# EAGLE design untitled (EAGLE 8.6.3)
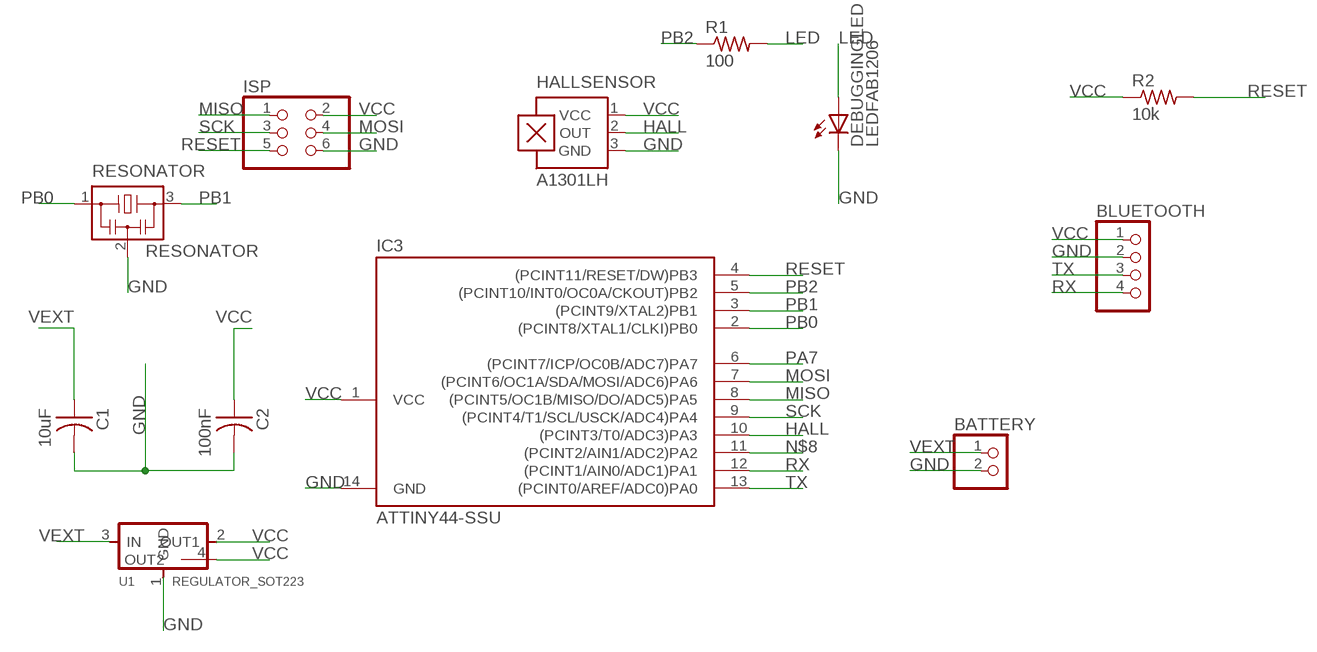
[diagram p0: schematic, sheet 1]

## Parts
BATTERY  PINHD-1X2  [1X02]
BLUETOOTH  PINHD-1X4  [1X04]
C1  10uF  CAP-US1206FAB  [C1206FAB]
C2  100nF  CAP-US1206FAB  [C1206FAB]
DEBUGGINGLED  LEDFAB1206  [LED1206FAB]
HALLSENSOR  A1301LH  [SOT23-W]
IC3  ATTINY44-SSU  [SOIC14]
ISP  PINHD-2X3-SMD  [2X03SMD]
R1  100  RES-US1206FAB  [R1206FAB]
R2  10k  RES-US1206FAB  [R1206FAB]
RESONATOR  RESONATOR  [EFOBM]
U1  REGULATOR_SOT223  [SOT223]

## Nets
GND: BATTERY.2 BLUETOOTH.2 C1.2 C2.2 DEBUGGINGLED.2(C) HALLSENSOR.3(GND) IC3.14(GND) ISP.6 RESONATOR.2 U1.1(GND)
HALL: HALLSENSOR.2(OUT) IC3.10((PCINT3/T0/ADC3)PA3)
LED: DEBUGGINGLED.1(A) R1.2
MISO: IC3.8((PCINT5/OC1B/MISO/DO/ADC5)PA5) ISP.1
MOSI: IC3.7((PCINT6/OC1A/SDA/MOSI/ADC6)PA6) ISP.4
N$8: IC3.11((PCINT2/AIN1/ADC2)PA2)
PA7: IC3.6((PCINT7/ICP/OC0B/ADC7)PA7)
PB0: IC3.2((PCINT8/XTAL1/CLKI)PB0) RESONATOR.1
PB1: IC3.3((PCINT9/XTAL2)PB1) RESONATOR.3
PB2: IC3.5((PCINT10/INT0/OC0A/CKOUT)PB2) R1.1
RESET: IC3.4((PCINT11/RESET/DW)PB3) ISP.5 R2.2
RX: BLUETOOTH.4 IC3.12((PCINT1/AIN0/ADC1)PA1)
SCK: IC3.9((PCINT4/T1/SCL/USCK/ADC4)PA4) ISP.3
TX: BLUETOOTH.3 IC3.13((PCINT0/AREF/ADC0)PA0)
VCC: BLUETOOTH.1 C2.1 HALLSENSOR.1(VCC) IC3.1(VCC) ISP.2 R2.1 U1.2(OUT1) U1.4(OUT2)
VEXT: BATTERY.1 C1.1 U1.3(IN)

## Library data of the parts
BATTERY = pinhead:PINHD-1X2: PIN HEADER
BLUETOOTH = pinhead:PINHD-1X4: PIN HEADER
C1 C2 = 01_fab:CAP-US
DEBUGGINGLED = 01_fab:LED: LED
HALLSENSOR = allegro:A13*?: Linear Hall Effect Sensor ICs Continuous-Time Ratiometric High-Temperature Operation Programmable Linear with Analog Output A1302 -Replacement- UGN3503 Source: http://www.allegromicro.com/en/Products/Part_Numbers/1301/1301.pdf http://www.allegromicro.com/en/Products/Part_Numbers/1321/1321.pdf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; MF: ALLEGRO MICROSYSTEMS, INC.; MPN: A1301ELHLT-T; OC_FARNELL: 1198084; OC_NEWARK: 31K6634
IC3 = 01_fab:ATTINY44
ISP = 01_fab:PINHD-2X3-SMD: PIN HEADER
R1 R2 = 01_fab:RES-US: Resistor (US Symbol)
RESONATOR = 01_fab:RESONATOR
U1 = 001_fab:REGULATOR_SOT223

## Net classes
0 default: clearance 0.205 mm

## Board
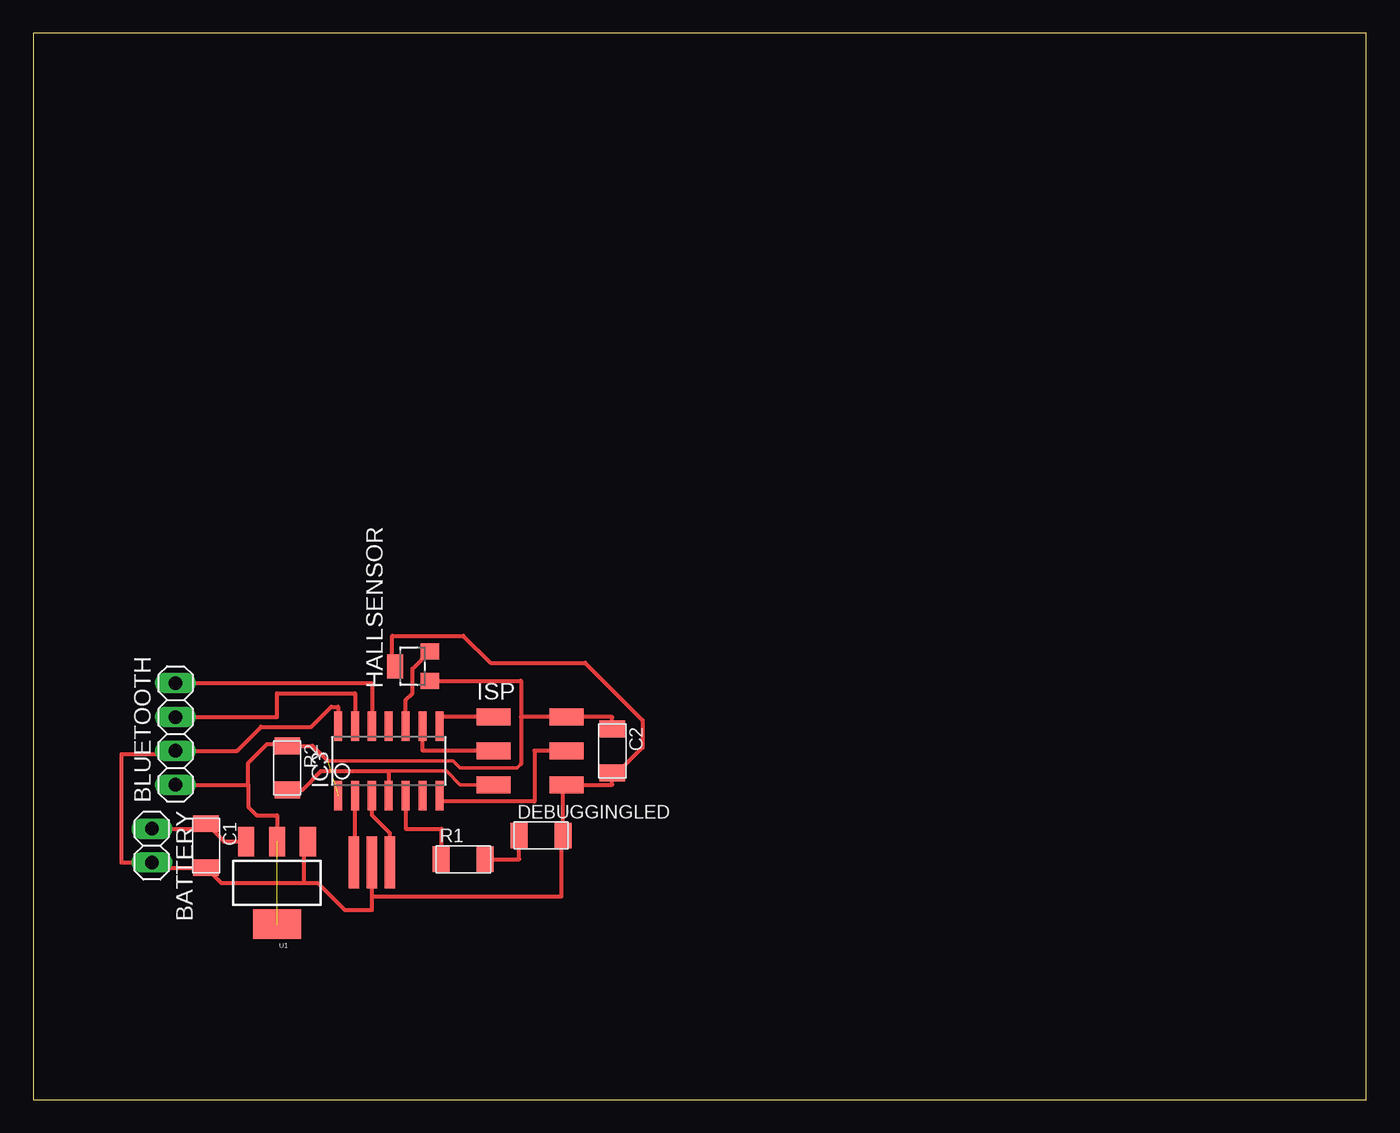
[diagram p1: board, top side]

Size 100 x 80 mm. Coordinates in mm from the lower left corner, seen from the top.
Outline: 0,0 100,0 100,80 0,80 0,0
Copper layers (1*16): Top 0.035mm / dielectric 1.5mm / Bottom 0.035mm
Design rules "default": minimum track width 6mil, minimum drill 0.35mm, track to track 6mil, track to pad 6mil, pad to pad 6mil, via to via 6mil, smd to smd 6mil, copper to edge 40mil, drill to drill 6mil, minimum pad ring 10mil, minimum via ring 8mil, stop-mask expansion 4mil, vias tented up to drill 0mil, thermal gap 10mil

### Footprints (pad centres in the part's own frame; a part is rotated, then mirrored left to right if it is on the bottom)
1X02 = drill 1.016 long: 1 -1.27,0; 2 1.27,0
1X04 = drill 1.016 long: 1 -3.81,0; 2 -1.27,0; 3 1.27,0; 4 3.81,0
C1206FAB = smd 1.27 x 1.905: 1 -1.651,0; 2 1.651,0
LED1206FAB = smd 1.27 x 1.905: 1 -1.651,0; 2 1.651,0
SOT23-W = smd 1.2 x 1.4: 1 -1.1,-1.3; 2 1.1,-1.3 | smd 1.8 x 1.2: 3 0,1.3
SOIC14 = smd 0.61 x 2.21: 1 -3.81,-2.603; 2 -2.54,-2.603; 3 -1.27,-2.603; 4 0,-2.603; 5 1.27,-2.603; 6 2.54,-2.603; 7 3.81,-2.603; 8 3.81,2.603; 9 2.54,2.603; 10 1.27,2.603; 11 0,2.603; 12 -1.27,2.603; 13 -2.54,2.603; 14 -3.81,2.603
2X03SMD = smd 2.54 x 1.27: 1 -2.54,2.54; 2 2.92,2.54; 3 -2.54,0; 4 2.92,0; 5 -2.54,-2.54; 6 2.92,-2.54
R1206FAB = smd 1.27 x 1.905: 1 -1.651,0; 2 1.651,0
EFOBM = smd 0.8 x 3.9: 1 -1.35,0; 2 0,0; 3 1.35,0
SOT223 = smd 1.219 x 2.235: 1 -2.311,-3.099; 2 0,-3.099; 3 2.311,-3.099 | smd 3.6 x 2.2: 4 0,3.099

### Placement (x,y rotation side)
BATTERY  8.89,19.05 270 top
BLUETOOTH  10.67,27.43 90 top
C1  12.95,19.05 270 top
C2  43.43,26.16 270 top
DEBUGGINGLED  38.1,19.81 0 top
HALLSENSOR  28.45,32.51 90 top
IC3  26.67,25.4 0 top
ISP  37.08,26.16 0 top
R1  32.26,18.03 0 top
R2  19.05,24.89 270 top
RESONATOR  25.4,17.78 0 top
U1  18.29,16.26 180 top

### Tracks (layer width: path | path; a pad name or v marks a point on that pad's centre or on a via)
GND
  Top 0.305: 43.43,24.13 43.43,23.62 ISP.6 39.75,23.62 DEBUGGINGLED.2 39.62,19.81 39.62,15.24 25.4,15.24 | 43.43,24.13 C2.2 | 25.4,15.24 RESONATOR.2 | IC3.14 22.86,29.46 22.35,29.46 20.86,27.97 17.09,27.97 15.28,26.16 BLUETOOTH.2 10.41,25.91 6.6,25.91 6.6,17.78 BATTERY.2 9.27,17.4 C1.2 14.1,16.26 20.32,16.26 | 20.32,16.26 20.32,19.07 U1.1 | 20.32,16.26 21.34,16.26 23.37,14.22 25.4,14.22 25.4,15.24 | HALLSENSOR.3 26.92,32.74 26.92,34.8 32.26,34.8 34.29,32.77 41.4,32.77 45.72,28.45 45.72,26.42 43.43,24.13
HALL
  Top 0.305: HALLSENSOR.2 28.45,32.31 28.45,30.48 27.94,29.97 IC3.10
LED
  Top 0.305: R1.2 36.45,18.03 DEBUGGINGLED.1
MISO
  Top 0.305: ISP.1 30.48,28.7 IC3.8
MOSI
  Top 0.305: ISP.4 37.59,26.16 37.59,22.35 30.48,22.35 IC3.7
PB0
  Top 0.305: RESONATOR.1 24.13,17.78 IC3.2
PB1
  Top 0.305: RESONATOR.3 26.75,19.99 25.4,21.34 IC3.3
PB2
  Top 0.305: IC3.5 27.94,20.32 30.61,20.32 R1.1
RESET
  Top 0.254: 26.67,24.64 30.99,24.64 32,23.62 ISP.5
  Top 0.305: R2.2 20.19,23.24 21.59,24.64 26.67,24.64 IC3.4
RX
  Top 0.305: IC3.12 25.4,31.24 BLUETOOTH.4
SCK
  Top 0.305: ISP.3 29.21,26.16 IC3.9
TX
  Top 0.305: IC3.13 24.13,30.48 18.29,30.48 18.29,28.7 BLUETOOTH.3
VCC  (2 unrouted)
  Top 0.254: 36.58,25.17 36.3,24.89 32,24.89 31.5,25.4 22.1,25.4
  Top 0.305: C2.1 43.43,28.7 ISP.2 36.58,28.7 | HALLSENSOR.1 36.58,31.41 36.58,28.7 | 36.58,28.7 36.58,25.17 | BLUETOOTH.1 16.13,23.62 | 16.13,23.62 16.13,25.27 17.53,26.67 18.92,26.67 R2.1 20.95,26.54 22.1,25.4 | 16.13,23.62 16.13,21.97 16.76,21.34 18.29,21.34 U1.2
VEXT
  Top 0.305: BATTERY.1 12.57,20.32 C1.1 14.3,19.36 U1.3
